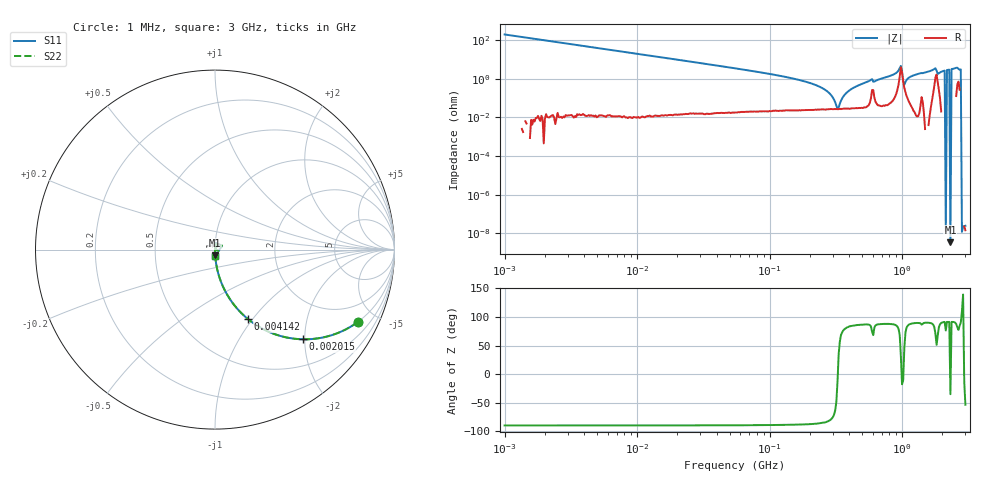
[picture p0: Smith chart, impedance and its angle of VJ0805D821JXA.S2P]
! VJ0805D821JXA
! DATE
! CORRECTED  DATA
# Hz  S  MA  R  50
!Freq	S11M	S11A	S21M	S21A	S12M	S12A	S22M	S22A
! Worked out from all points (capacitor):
!   401 points, 1 MHz to 3 GHz, reference 50 ohm
!   read as one part in series: C = 807 pF near 1.041 MHz
!   lowest |Z| = 3.45 nohm at 2.313 GHz (marker M1)
!   series resonance near 326.8 MHz, so ESL is about 290 pH
!   S11 on the Smith chart (normalised r, x): 1 MHz: 1.00, -3.94; 2.015 MHz: 1.00, -1.96; 4.142 MHz: 1.00, -0.95; 3 GHz: 1.00, -0.07
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1000000  0.892 -26.9  0.4522 63.1  0.4522 63.1  0.892 -26.9
2014875  0.6995 -45.6  0.7146 44.4  0.7146 44.4  0.6995 -45.6
3823119  0.4584 -62.7  0.8886 27.3  0.8886 27.3  0.4584 -62.7
4141799  0.4298 -64.5  0.9028 25.5  0.9028 25.5  0.4298 -64.5
1.461624e7  0.1334 -82.3  0.9909 7.7  0.9909 7.7  0.1334 -82.3
5.587962e7  0.0342 -87.7  0.9992 2.0  0.9992 2.0  0.0342 -87.7
2.094008e8  0.005555 -87.2  0.9997 0.3  0.9997 0.3  0.005555 -87.2
2.771263e8  0.002015 -82.3  0.9997 0.1  0.9997 0.1  0.002015 -82.3
3.252521e8  0.0002764 -12.6  0.9997 0.0  0.9997 0.0  0.0002764 -12.6
3.385367e8  0.0005145 56.9  0.9997 -0.0  0.9997 -0.0  0.0005145 56.9
3.741707e8  0.001683 80.0  0.9997 -0.1  0.9997 -0.1  0.001683 80.0
4.304467e8  0.003455 84.9  0.9997 -0.2  0.9997 -0.2  0.003455 84.9
5.696638e8  0.008058 85.6  0.9994 -0.5  0.9994 -0.5  0.008058 85.6
6.296259e8  0.007818 84.9  0.9993 -0.4  0.9993 -0.4  0.007818 84.9
8.005644e8  0.01374 87.1  0.9994 -0.8  0.9994 -0.8  0.01374 87.1
9.585869e8  0.03518 66.2  0.9863 -1.9  0.9863 -1.9  0.03518 66.2
1.059487e9  0.006873 73.0  0.998 -0.4  0.998 -0.4  0.006873 73.0
1.194682e9  0.01426 88.0  0.9996 -0.8  0.9996 -0.8  0.01426 88.0
1.712864e9  0.02945 85.0  0.9979 -1.7  0.9979 -1.7  0.02945 85.0
1.931433e9  0.02125 86.3  0.9988 -1.2  0.9988 -1.2  0.02125 86.3
2.312676e9  0.03081 -89.9  1.001 -1.8  1.001 -1.8  0.03081 -89.9
3e9  0.03555 -87.8  1.002 -2.0  1.002 -2.0  0.03555 -87.8
